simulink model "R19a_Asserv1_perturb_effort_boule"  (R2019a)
settings: Solver=ode15s  StartTime=0.0  StopTime=1  RelTol=1e-3  EnableMultiTasking=on
undefined symbols (not defined in the file): deg, kg, m, manette1_Défaut_sldprt, manette2_Défaut_sldprt, mm, N, rad, s, sigbuilder_block, STL, X, Y, Z
libraries: sm_lib x460, fl_lib x45, nesl_utility x23, simulink x3
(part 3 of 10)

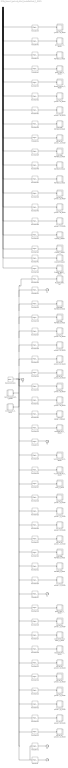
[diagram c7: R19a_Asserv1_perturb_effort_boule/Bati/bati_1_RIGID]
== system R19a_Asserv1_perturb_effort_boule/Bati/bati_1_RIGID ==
  CACHE_1_RIGID : Subsystem
  CACHE_2_RIGID : Subsystem
  CACHE_3_RIGID : Subsystem
  CARTER_ARRIERE_1_RIGID : Subsystem
  CARTE_HEXAGONALE_1_RIGID : Subsystem
  FIXATION_MOTEUR_1_RIGID : Subsystem
  FIXATION_MOTEUR_2_RIGID : Subsystem
  FIXATION_MOTEUR_3_RIGID : Subsystem
  FIXATION_MOTEUR_4_RIGID : Subsystem
  FIXATION_MOTEUR_5_RIGID : Subsystem
  FIXATION_MOTEUR_6_RIGID : Subsystem
  MOTEUR_1_RIGID : Subsystem
  MOTEUR_2_RIGID : Subsystem
  MOTEUR_3_RIGID : Subsystem
  PLAQUE_NOM_1_RIGID : Subsystem
  PLAQUE_NOM_SET : Subsystem
  ReferenceFrame : sm_lib/Frames and Transforms/Reference Frame
  Rondelle_M4_1_RIGID : Subsystem
  Rondelle_M4_2_RIGID : Subsystem
  Transform : sm_lib/Frames and Transforms/Rigid Transform  TranslationMethod=Cartesian  TranslationStandardOffset=0  TranslationLengthUnit=mm  TranslationStandardAxis=+Z  TranslationCartesianOffset=[-67.982453021745741 154.13917308955064 38.499999999999979]  TranslationROffset=0  TranslationROffsetUnits=m  TranslationZOffset=0  TranslationZOffsetUnits=m  TranslationThetaOffset=0  TranslationThetaOffsetUnits=deg  RotationMethod=ArbitraryAxis  RotationAngleUnits=rad  RotationStandardAxis=+Z  RotationAngle=2.2576709855630241  RotationArbitraryAxis=[-0.47317816576134769 -0.62293756647304832 0.62293756647304788]  FollAlignAxisA=+X  BaseAlignAxisA=+Y  FollAlignAxisB=+Y  BaseAlignAxisB=+Z  RotationSequenceAxes=FollowerAxes  RotationSequence=XYX  RotationSequenceAngles=[0 0 0]  RotationSequenceAnglesUnits=deg  RotationMatrix=[1 0 0; 0 1 0; 0 0 1]
  Transform1 : sm_lib/Frames and Transforms/Rigid Transform  TranslationMethod=Cartesian  TranslationStandardOffset=0  TranslationLengthUnit=mm  TranslationStandardAxis=+Z  TranslationCartesianOffset=[67.670238338594061 154.67994478363838 38.499999999999979]  TranslationROffset=0  TranslationROffsetUnits=m  TranslationZOffset=0  TranslationZOffsetUnits=m  TranslationThetaOffset=0  TranslationThetaOffsetUnits=deg  RotationMethod=ArbitraryAxis  RotationAngleUnits=rad  RotationStandardAxis=+Z  RotationAngle=2.2455218567975841  RotationArbitraryAxis=[-0.62007686508407689 -0.48063433374552811 -0.62007686508407622]  FollAlignAxisA=+X  BaseAlignAxisA=+Y  FollAlignAxisB=+Y  BaseAlignAxisB=+Z  RotationSequenceAxes=FollowerAxes  RotationSequence=XYX  RotationSequenceAngles=[0 0 0]  RotationSequenceAnglesUnits=deg  RotationMatrix=[1 0 0; 0 1 0; 0 0 1]
  Transform10 : sm_lib/Frames and Transforms/Rigid Transform  TranslationMethod=Cartesian  TranslationStandardOffset=0  TranslationLengthUnit=mm  TranslationStandardAxis=+Z  TranslationCartesianOffset=[-21.302011487444762 191.53150356202462 36.100000000000051]  TranslationROffset=0  TranslationROffsetUnits=m  TranslationZOffset=0  TranslationZOffsetUnits=m  TranslationThetaOffset=0  TranslationThetaOffsetUnits=deg  RotationMethod=ArbitraryAxis  RotationAngleUnits=rad  RotationStandardAxis=+Z  RotationAngle=1.5874169403231204  RotationArbitraryAxis=[0.12785986324311854 -0.98351599414696989 0.12785986324311688]  FollAlignAxisA=+X  BaseAlignAxisA=+Y  FollAlignAxisB=+Y  BaseAlignAxisB=+Z  RotationSequenceAxes=FollowerAxes  RotationSequence=XYX  RotationSequenceAngles=[0 0 0]  RotationSequenceAnglesUnits=deg  RotationMatrix=[1 0 0; 0 1 0; 0 0 1]
  Transform11 : sm_lib/Frames and Transforms/Rigid Transform  TranslationMethod=Cartesian  TranslationStandardOffset=0  TranslationLengthUnit=mm  TranslationStandardAxis=+Z  TranslationCartesianOffset=[-8.6943864691458312 146.25405010671241 36.099999999999994]  TranslationROffset=0  TranslationROffsetUnits=m  TranslationZOffset=0  TranslationZOffsetUnits=m  TranslationThetaOffset=0  TranslationThetaOffsetUnits=deg  RotationMethod=ArbitraryAxis  RotationAngleUnits=rad  RotationStandardAxis=+Z  RotationAngle=2.557922199918194  RotationArbitraryAxis=[0.67444507075713422 -0.30041253812517366 0.67444507075713389]  FollAlignAxisA=+X  BaseAlignAxisA=+Y  FollAlignAxisB=+Y  BaseAlignAxisB=+Z  RotationSequenceAxes=FollowerAxes  RotationSequence=XYX  RotationSequenceAngles=[0 0 0]  RotationSequenceAnglesUnits=deg  RotationMatrix=[1 0 0; 0 1 0; 0 0 1]
  Transform12 : sm_lib/Frames and Transforms/Rigid Transform  TranslationMethod=Cartesian  TranslationStandardOffset=0  TranslationLengthUnit=mm  TranslationStandardAxis=+Z  TranslationCartesianOffset=[31.197488247191473 107.27753449924363 36.099999999999994]  TranslationROffset=0  TranslationROffsetUnits=m  TranslationZOffset=0  TranslationZOffsetUnits=m  TranslationThetaOffset=0  TranslationThetaOffsetUnits=deg  RotationMethod=ArbitraryAxis  RotationAngleUnits=rad  RotationStandardAxis=+Z  RotationAngle=1.5816892610060764  RotationArbitraryAxis=[0.10380436397422958 -0.98916596587216399 0.10380436397423064]  FollAlignAxisA=+X  BaseAlignAxisA=+Y  FollAlignAxisB=+Y  BaseAlignAxisB=+Z  RotationSequenceAxes=FollowerAxes  RotationSequence=XYX  RotationSequenceAngles=[0 0 0]  RotationSequenceAnglesUnits=deg  RotationMatrix=[1 0 0; 0 1 0; 0 0 1]
  Transform13 : sm_lib/Frames and Transforms/Rigid Transform  TranslationMethod=Cartesian  TranslationStandardOffset=0  TranslationLengthUnit=mm  TranslationStandardAxis=+Z  TranslationCartesianOffset=[-32.1104315373926 141.51053427005223 49.100000000000001]  TranslationROffset=0  TranslationROffsetUnits=m  TranslationZOffset=0  TranslationZOffsetUnits=m  TranslationThetaOffset=0  TranslationThetaOffsetUnits=deg  RotationMethod=ArbitraryAxis  RotationAngleUnits=rad  RotationStandardAxis=+Z  RotationAngle=2.4188584057763718  RotationArbitraryAxis=[-0.65465367070797598 -0.37796447300923064 -0.6546536707079762]  FollAlignAxisA=+X  BaseAlignAxisA=+Y  FollAlignAxisB=+Y  BaseAlignAxisB=+Z  RotationSequenceAxes=FollowerAxes  RotationSequence=XYX  RotationSequenceAngles=[0 0 0]  RotationSequenceAnglesUnits=deg  RotationMatrix=[1 0 0; 0 1 0; 0 0 1]
  Transform14 : sm_lib/Frames and Transforms/Rigid Transform  TranslationMethod=Cartesian  TranslationStandardOffset=0  TranslationLengthUnit=mm  TranslationStandardAxis=+Z  TranslationCartesianOffset=[76.71272566730876 95.557331318822435 36.100000000000051]  TranslationROffset=0  TranslationROffsetUnits=m  TranslationZOffset=0  TranslationZOffsetUnits=m  TranslationThetaOffset=0  TranslationThetaOffsetUnits=deg  RotationMethod=ArbitraryAxis  RotationAngleUnits=rad  RotationStandardAxis=+Z  RotationAngle=2.253606277940353  RotationArbitraryAxis=[-0.62198874395633519 -0.47566795643940651 -0.62198874395633508]  FollAlignAxisA=+X  BaseAlignAxisA=+Y  FollAlignAxisB=+Y  BaseAlignAxisB=+Z  RotationSequenceAxes=FollowerAxes  RotationSequence=XYX  RotationSequenceAngles=[0 0 0]  RotationSequenceAnglesUnits=deg  RotationMatrix=[1 0 0; 0 1 0; 0 0 1]
  Transform15 : sm_lib/Frames and Transforms/Rigid Transform  TranslationMethod=Cartesian  TranslationStandardOffset=0  TranslationLengthUnit=mm  TranslationStandardAxis=+Z  TranslationCartesianOffset=[39.05251803832482 137.78242766379034 36.099999999999966]  TranslationROffset=0  TranslationROffsetUnits=m  TranslationZOffset=0  TranslationZOffsetUnits=m  TranslationThetaOffset=0  TranslationThetaOffsetUnits=deg  RotationMethod=ArbitraryAxis  RotationAngleUnits=rad  RotationStandardAxis=+Z  RotationAngle=2.1395291955010958  RotationArbitraryAxis=[-0.59164485304725056 -0.54764289069191197 -0.59164485304725156]  FollAlignAxisA=+X  BaseAlignAxisA=+Y  FollAlignAxisB=+Y  BaseAlignAxisB=+Z  RotationSequenceAxes=FollowerAxes  RotationSequence=XYX  RotationSequenceAngles=[0 0 0]  RotationSequenceAnglesUnits=deg  RotationMatrix=[1 0 0; 0 1 0; 0 0 1]
  Transform16 : sm_lib/Frames and Transforms/Rigid Transform  TranslationMethod=Cartesian  TranslationStandardOffset=0  TranslationLengthUnit=mm  TranslationStandardAxis=+Z  TranslationCartesianOffset=[-9.8750000000000053 1.2000000000000066 14.050000000000008]  TranslationROffset=0  TranslationROffsetUnits=m  TranslationZOffset=0  TranslationZOffsetUnits=m  TranslationThetaOffset=0  TranslationThetaOffsetUnits=deg  RotationMethod=ArbitraryAxis  RotationAngleUnits=rad  RotationStandardAxis=+Z  RotationAngle=0.1305039651717789  RotationArbitraryAxis=[1.6038157489539324e-15 1 -1.2797090690177757e-15]  FollAlignAxisA=+X  BaseAlignAxisA=+Y  FollAlignAxisB=+Y  BaseAlignAxisB=+Z  RotationSequenceAxes=FollowerAxes  RotationSequence=XYX  RotationSequenceAngles=[0 0 0]  RotationSequenceAnglesUnits=deg  RotationMatrix=[1 0 0; 0 1 0; 0 0 1]
  Transform17 : sm_lib/Frames and Transforms/Rigid Transform  TranslationMethod=Cartesian  TranslationStandardOffset=0  TranslationLengthUnit=mm  TranslationStandardAxis=+Z  TranslationCartesianOffset=[0 115.25000000000001 16.899999999999999]  TranslationROffset=0  TranslationROffsetUnits=m  TranslationZOffset=0  TranslationZOffsetUnits=m  TranslationThetaOffset=0  TranslationThetaOffsetUnits=deg  RotationMethod=ArbitraryAxis  RotationAngleUnits=rad  RotationStandardAxis=+Z  RotationAngle=3.1415926535897931  RotationArbitraryAxis=[-0.14780941112961105 0.98901586336191671 0]  FollAlignAxisA=+X  BaseAlignAxisA=+Y  FollAlignAxisB=+Y  BaseAlignAxisB=+Z  RotationSequenceAxes=FollowerAxes  RotationSequence=XYX  RotationSequenceAngles=[0 0 0]  RotationSequenceAnglesUnits=deg  RotationMatrix=[1 0 0; 0 1 0; 0 0 1]
  Transform18 : sm_lib/Frames and Transforms/Rigid Transform  TranslationMethod=Cartesian  TranslationStandardOffset=0  TranslationLengthUnit=mm  TranslationStandardAxis=+Z  TranslationCartesianOffset=[0 115.25000000000001 -1.799999999999996]  TranslationROffset=0  TranslationROffsetUnits=m  TranslationZOffset=0  TranslationZOffsetUnits=m  TranslationThetaOffset=0  TranslationThetaOffsetUnits=deg  RotationMethod=ArbitraryAxis  RotationAngleUnits=rad  RotationStandardAxis=+Z  RotationAngle=3.1415926535897909  RotationArbitraryAxis=[-0.70710678118654757 -1.2168216554799258e-15 -0.70710678118654746]  FollAlignAxisA=+X  BaseAlignAxisA=+Y  FollAlignAxisB=+Y  BaseAlignAxisB=+Z  RotationSequenceAxes=FollowerAxes  RotationSequence=XYX  RotationSequenceAngles=[0 0 0]  RotationSequenceAnglesUnits=deg  RotationMatrix=[1 0 0; 0 1 0; 0 0 1]
  Transform19 : sm_lib/Frames and Transforms/Rigid Transform  TranslationMethod=Cartesian  TranslationStandardOffset=0  TranslationLengthUnit=mm  TranslationStandardAxis=+Z  TranslationCartesianOffset=[-5.4923264138695282 106.15877278095202 52.900000000000013]  TranslationROffset=0  TranslationROffsetUnits=m  TranslationZOffset=0  TranslationZOffsetUnits=m  TranslationThetaOffset=0  TranslationThetaOffsetUnits=deg  RotationMethod=ArbitraryAxis  RotationAngleUnits=rad  RotationStandardAxis=+Z  RotationAngle=3.1415926535897931  RotationArbitraryAxis=[-0.62251463663761875 0.78260815685241447 9.5278235956943858e-17]  FollAlignAxisA=+X  BaseAlignAxisA=+Y  FollAlignAxisB=+Y  BaseAlignAxisB=+Z  RotationSequenceAxes=FollowerAxes  RotationSequence=XYX  RotationSequenceAngles=[0 0 0]  RotationSequenceAnglesUnits=deg  RotationMatrix=[1 0 0; 0 1 0; 0 0 1]
  Transform2 : sm_lib/Frames and Transforms/Rigid Transform  TranslationMethod=Cartesian  TranslationStandardOffset=0  TranslationLengthUnit=mm  TranslationStandardAxis=+Z  TranslationCartesianOffset=[0.3122146831511497 36.930882126810701 38.499999999999979]  TranslationROffset=0  TranslationROffsetUnits=m  TranslationZOffset=0  TranslationZOffsetUnits=m  TranslationThetaOffset=0  TranslationThetaOffsetUnits=deg  RotationMethod=ArbitraryAxis  RotationAngleUnits=rad  RotationStandardAxis=+Z  RotationAngle=1.7212826903554606  RotationArbitraryAxis=[0.85979818153437826 0.36107276761767659 0.36107276761767548]  FollAlignAxisA=+X  BaseAlignAxisA=+Y  FollAlignAxisB=+Y  BaseAlignAxisB=+Z  RotationSequenceAxes=FollowerAxes  RotationSequence=XYX  RotationSequenceAngles=[0 0 0]  RotationSequenceAnglesUnits=deg  RotationMatrix=[1 0 0; 0 1 0; 0 0 1]
  Transform20 : sm_lib/Frames and Transforms/Rigid Transform  TranslationMethod=Cartesian  TranslationStandardOffset=0  TranslationLengthUnit=mm  TranslationStandardAxis=+Z  TranslationCartesianOffset=[-6.6870740261211532 74.311283427110965 49.100000000000001]  TranslationROffset=0  TranslationROffsetUnits=m  TranslationZOffset=0  TranslationZOffsetUnits=m  TranslationThetaOffset=0  TranslationThetaOffsetUnits=deg  RotationMethod=ArbitraryAxis  RotationAngleUnits=rad  RotationStandardAxis=+Z  RotationAngle=1.5707963267948968  RotationArbitraryAxis=[-0 -1 -1.8723979605913744e-16]  FollAlignAxisA=+X  BaseAlignAxisA=+Y  FollAlignAxisB=+Y  BaseAlignAxisB=+Z  RotationSequenceAxes=FollowerAxes  RotationSequence=XYX  RotationSequenceAngles=[0 0 0]  RotationSequenceAnglesUnits=deg  RotationMatrix=[1 0 0; 0 1 0; 0 0 1]
  Transform21 : sm_lib/Frames and Transforms/Rigid Transform  TranslationMethod=Cartesian  TranslationStandardOffset=0  TranslationLengthUnit=mm  TranslationStandardAxis=+Z  TranslationCartesianOffset=[-16.466410454294302 53.38468832772007 38.500000000000007]  TranslationROffset=0  TranslationROffsetUnits=m  TranslationZOffset=0  TranslationZOffsetUnits=m  TranslationThetaOffset=0  TranslationThetaOffsetUnits=deg  RotationMethod=ArbitraryAxis  RotationAngleUnits=rad  RotationStandardAxis=+Z  RotationAngle=2.5869353710023297  RotationArbitraryAxis=[-0.28466429222446077 0.67785184248932562 -0.6778518424893254]  FollAlignAxisA=+X  BaseAlignAxisA=+Y  FollAlignAxisB=+Y  BaseAlignAxisB=+Z  RotationSequenceAxes=FollowerAxes  RotationSequence=XYX  RotationSequenceAngles=[0 0 0]  RotationSequenceAnglesUnits=deg  RotationMatrix=[1 0 0; 0 1 0; 0 0 1]
  Transform22 : sm_lib/Frames and Transforms/Rigid Transform  TranslationMethod=Cartesian  TranslationStandardOffset=0  TranslationLengthUnit=mm  TranslationStandardAxis=+Z  TranslationCartesianOffset=[-38.956907978955229 75.439790256598585 38.500000000000028]  TranslationROffset=0  TranslationROffsetUnits=m  TranslationZOffset=0  TranslationZOffsetUnits=m  TranslationThetaOffset=0  TranslationThetaOffsetUnits=deg  RotationMethod=ArbitraryAxis  RotationAngleUnits=rad  RotationStandardAxis=+Z  RotationAngle=2.5869353710023297  RotationArbitraryAxis=[-0.28466429222446077 0.67785184248932562 -0.67785184248932528]  FollAlignAxisA=+X  BaseAlignAxisA=+Y  FollAlignAxisB=+Y  BaseAlignAxisB=+Z  RotationSequenceAxes=FollowerAxes  RotationSequence=XYX  RotationSequenceAngles=[0 0 0]  RotationSequenceAnglesUnits=deg  RotationMatrix=[1 0 0; 0 1 0; 0 0 1]
  Transform23 : sm_lib/Frames and Transforms/Rigid Transform  TranslationMethod=Cartesian  TranslationStandardOffset=0  TranslationLengthUnit=mm  TranslationStandardAxis=+Z  TranslationCartesianOffset=[-32.920216655203667 36.606063190274597 36.100000000000037]  TranslationROffset=0  TranslationROffsetUnits=m  TranslationZOffset=0  TranslationZOffsetUnits=m  TranslationThetaOffset=0  TranslationThetaOffsetUnits=deg  RotationMethod=ArbitraryAxis  RotationAngleUnits=rad  RotationStandardAxis=+Z  RotationAngle=2.1079572963404796  RotationArbitraryAxis=[0.58180115951651357 -0.56834392894662011 0.58180115951651357]  FollAlignAxisA=+X  BaseAlignAxisA=+Y  FollAlignAxisB=+Y  BaseAlignAxisB=+Z  RotationSequenceAxes=FollowerAxes  RotationSequence=XYX  RotationSequenceAngles=[0 0 0]  RotationSequenceAnglesUnits=deg  RotationMatrix=[1 0 0; 0 1 0; 0 0 1]
  Transform24 : sm_lib/Frames and Transforms/Rigid Transform  TranslationMethod=Cartesian  TranslationStandardOffset=0  TranslationLengthUnit=mm  TranslationStandardAxis=+Z  TranslationCartesianOffset=[-55.410714179864605 58.661165119153118 36.100000000000051]  TranslationROffset=0  TranslationROffsetUnits=m  TranslationZOffset=0  TranslationZOffsetUnits=m  TranslationThetaOffset=0  TranslationThetaOffsetUnits=deg  RotationMethod=ArbitraryAxis  RotationAngleUnits=rad  RotationStandardAxis=+Z  RotationAngle=2.5913633997650876  RotationArbitraryAxis=[0.67835179231251819 -0.28227237153641171 0.67835179231251697]  FollAlignAxisA=+X  BaseAlignAxisA=+Y  FollAlignAxisB=+Y  BaseAlignAxisB=+Z  RotationSequenceAxes=FollowerAxes  RotationSequence=XYX  RotationSequenceAngles=[0 0 0]  RotationSequenceAnglesUnits=deg  RotationMatrix=[1 0 0; 0 1 0; 0 0 1]
  Transform25 : sm_lib/Frames and Transforms/Rigid Transform  TranslationMethod=Cartesian  TranslationStandardOffset=0  TranslationLengthUnit=mm  TranslationStandardAxis=+Z  TranslationCartesianOffset=[-0.012604253384927124 70.163313465165515 36.099999999999966]  TranslationROffset=0  TranslationROffsetUnits=m  TranslationZOffset=0  TranslationZOffsetUnits=m  TranslationThetaOffset=0  TranslationThetaOffsetUnits=deg  RotationMethod=ArbitraryAxis  RotationAngleUnits=rad  RotationStandardAxis=+Z  RotationAngle=2.7200049334585095  RotationArbitraryAxis=[0.6907299635194234 -0.21397250990001554 0.6907299635194234]  FollAlignAxisA=+X  BaseAlignAxisA=+Y  FollAlignAxisB=+Y  BaseAlignAxisB=+Z  RotationSequenceAxes=FollowerAxes  RotationSequence=XYX  RotationSequenceAngles=[0 0 0]  RotationSequenceAnglesUnits=deg  RotationMatrix=[1 0 0; 0 1 0; 0 0 1]
  Transform26 : sm_lib/Frames and Transforms/Rigid Transform  TranslationMethod=Cartesian  TranslationStandardOffset=0  TranslationLengthUnit=mm  TranslationStandardAxis=+Z  TranslationCartesianOffset=[-22.503101778045874 92.21841539404403 36.099999999999994]  TranslationROffset=0  TranslationROffsetUnits=m  TranslationZOffset=0  TranslationZOffsetUnits=m  TranslationThetaOffset=0  TranslationThetaOffsetUnits=deg  RotationMethod=ArbitraryAxis  RotationAngleUnits=rad  RotationStandardAxis=+Z  RotationAngle=2.2845314039372839  RotationArbitraryAxis=[-0.62900467206978528 -0.4568437862429186 -0.62900467206978417]  FollAlignAxisA=+X  BaseAlignAxisA=+Y  FollAlignAxisB=+Y  BaseAlignAxisB=+Z  RotationSequenceAxes=FollowerAxes  RotationSequence=XYX  RotationSequenceAngles=[0 0 0]  RotationSequenceAnglesUnits=deg  RotationMatrix=[1 0 0; 0 1 0; 0 0 1]
  Transform27 : sm_lib/Frames and Transforms/Rigid Transform  TranslationMethod=Cartesian  TranslationStandardOffset=0  TranslationLengthUnit=mm  TranslationStandardAxis=+Z  TranslationCartesianOffset=[0 -1.5000000000000151 37.700000000000003]  TranslationROffset=0  TranslationROffsetUnits=m  TranslationZOffset=0  TranslationZOffsetUnits=m  TranslationThetaOffset=0  TranslationThetaOffsetUnits=deg  RotationMethod=ArbitraryAxis  RotationAngleUnits=rad  RotationStandardAxis=+Z  RotationAngle=1.5707963267948961  RotationArbitraryAxis=[-1 0 0]  FollAlignAxisA=+X  BaseAlignAxisA=+Y  FollAlignAxisB=+Y  BaseAlignAxisB=+Z  RotationSequenceAxes=FollowerAxes  RotationSequence=XYX  RotationSequenceAngles=[0 0 0]  RotationSequenceAnglesUnits=deg  RotationMatrix=[1 0 0; 0 1 0; 0 0 1]
  Transform28 : sm_lib/Frames and Transforms/Rigid Transform  TranslationMethod=Cartesian  TranslationStandardOffset=0  TranslationLengthUnit=mm  TranslationStandardAxis=+Z  TranslationCartesianOffset=[9.8750000000000089 31.199999999999992 14.050000000000008]  TranslationROffset=0  TranslationROffsetUnits=m  TranslationZOffset=0  TranslationZOffsetUnits=m  TranslationThetaOffset=0  TranslationThetaOffsetUnits=deg  RotationMethod=ArbitraryAxis  RotationAngleUnits=rad  RotationStandardAxis=+Z  RotationAngle=2.773492570857111  RotationArbitraryAxis=[0.18615678789738549 -0.69474659060686594 0.69474659060686572]  FollAlignAxisA=+X  BaseAlignAxisA=+Y  FollAlignAxisB=+Y  BaseAlignAxisB=+Z  RotationSequenceAxes=FollowerAxes  RotationSequence=XYX  RotationSequenceAngles=[0 0 0]  RotationSequenceAnglesUnits=deg  RotationMatrix=[1 0 0; 0 1 0; 0 0 1]
  Transform29 : sm_lib/Frames and Transforms/Rigid Transform  TranslationMethod=Cartesian  TranslationStandardOffset=0  TranslationLengthUnit=mm  TranslationStandardAxis=+Z  TranslationCartesianOffset=[-9.8750000000000053 31.199999999999992 14.050000000000008]  TranslationROffset=0  TranslationROffsetUnits=m  TranslationZOffset=0  TranslationZOffsetUnits=m  TranslationThetaOffset=0  TranslationThetaOffsetUnits=deg  RotationMethod=ArbitraryAxis  RotationAngleUnits=rad  RotationStandardAxis=+Z  RotationAngle=2.773492570857111  RotationArbitraryAxis=[0.18615678789738549 -0.69474659060686594 0.69474659060686572]  FollAlignAxisA=+X  BaseAlignAxisA=+Y  FollAlignAxisB=+Y  BaseAlignAxisB=+Z  RotationSequenceAxes=FollowerAxes  RotationSequence=XYX  RotationSequenceAngles=[0 0 0]  RotationSequenceAnglesUnits=deg  RotationMatrix=[1 0 0; 0 1 0; 0 0 1]
  Transform3 : sm_lib/Frames and Transforms/Rigid Transform  TranslationMethod=Cartesian  TranslationStandardOffset=0  TranslationLengthUnit=mm  TranslationStandardAxis=+Z  TranslationCartesianOffset=[-106.82639785458468 167.86430788780581 99.318100970001225]  TranslationROffset=0  TranslationROffsetUnits=m  TranslationZOffset=0  TranslationZOffsetUnits=m  TranslationThetaOffset=0  TranslationThetaOffsetUnits=deg  RotationMethod=ArbitraryAxis  RotationAngleUnits=rad  RotationStandardAxis=+Z  RotationAngle=1.7212826903554632  RotationArbitraryAxis=[0.85979818153438259 0.36107276761767909 0.36107276761766205]  FollAlignAxisA=+X  BaseAlignAxisA=+Y  FollAlignAxisB=+Y  BaseAlignAxisB=+Z  RotationSequenceAxes=FollowerAxes  RotationSequence=XYX  RotationSequenceAngles=[0 0 0]  RotationSequenceAnglesUnits=deg  RotationMatrix=[1 0 0; 0 1 0; 0 0 1]
  Transform30 : sm_lib/Frames and Transforms/Rigid Transform  TranslationMethod=Cartesian  TranslationStandardOffset=0  TranslationLengthUnit=mm  TranslationStandardAxis=+Z  TranslationCartesianOffset=[9.8750000000000089 2.0000000000000018 14.050000000000008]  TranslationROffset=0  TranslationROffsetUnits=m  TranslationZOffset=0  TranslationZOffsetUnits=m  TranslationThetaOffset=0  TranslationThetaOffsetUnits=deg  RotationMethod=ArbitraryAxis  RotationAngleUnits=rad  RotationStandardAxis=+Z  RotationAngle=3.1415926535897931  RotationArbitraryAxis=[-0.99787184465383982 -0 0.065205687230048659]  FollAlignAxisA=+X  BaseAlignAxisA=+Y  FollAlignAxisB=+Y  BaseAlignAxisB=+Z  RotationSequenceAxes=FollowerAxes  RotationSequence=XYX  RotationSequenceAngles=[0 0 0]  RotationSequenceAnglesUnits=deg  RotationMatrix=[1 0 0; 0 1 0; 0 0 1]
  Transform31 : sm_lib/Frames and Transforms/Rigid Transform  TranslationMethod=None  TranslationStandardOffset=0  TranslationLengthUnit=m  TranslationStandardAxis=+Z  TranslationCartesianOffset=[0 0 0]  TranslationROffset=0  TranslationROffsetUnits=m  TranslationZOffset=0  TranslationZOffsetUnits=m  TranslationThetaOffset=0  TranslationThetaOffsetUnits=deg  RotationMethod=ArbitraryAxis  RotationAngleUnits=rad  RotationStandardAxis=+Z  RotationAngle=3.1415926535897931  RotationArbitraryAxis=[0 1 0]  FollAlignAxisA=+X  BaseAlignAxisA=+Y  FollAlignAxisB=+Y  BaseAlignAxisB=+Z  RotationSequenceAxes=FollowerAxes  RotationSequence=XYX  RotationSequenceAngles=[0 0 0]  RotationSequenceAnglesUnits=deg  RotationMatrix=[1 0 0; 0 1 0; 0 0 1]
  Transform32 : sm_lib/Frames and Transforms/Rigid Transform  TranslationMethod=Cartesian  TranslationStandardOffset=0  TranslationLengthUnit=mm  TranslationStandardAxis=+Z  TranslationCartesianOffset=[78.177113545509911 88.894999319852587 19.199999999999996]  TranslationROffset=0  TranslationROffsetUnits=m  TranslationZOffset=0  TranslationZOffsetUnits=m  TranslationThetaOffset=0  TranslationThetaOffsetUnits=deg  RotationMethod=ArbitraryAxis  RotationAngleUnits=rad  RotationStandardAxis=+Z  RotationAngle=1.6591931073504684  RotationArbitraryAxis=[-0.28481620059537222 -0.91529201010214944 -0.28481620059537222]  FollAlignAxisA=+X  BaseAlignAxisA=+Y  FollAlignAxisB=+Y  BaseAlignAxisB=+Z  RotationSequenceAxes=FollowerAxes  RotationSequence=XYX  RotationSequenceAngles=[0 0 0]  RotationSequenceAnglesUnits=deg  RotationMatrix=[1 0 0; 0 1 0; 0 0 1]
  Transform33 : sm_lib/Frames and Transforms/Rigid Transform  TranslationMethod=Cartesian  TranslationStandardOffset=0  TranslationLengthUnit=mm  TranslationStandardAxis=+Z  TranslationCartesianOffset=[56.590549141302901 55.218676943733961 19.199999999999996]  TranslationROffset=0  TranslationROffsetUnits=m  TranslationZOffset=0  TranslationZOffsetUnits=m  TranslationThetaOffset=0  TranslationThetaOffsetUnits=deg  RotationMethod=ArbitraryAxis  RotationAngleUnits=rad  RotationStandardAxis=+Z  RotationAngle=1.5707963267948968  RotationArbitraryAxis=[-0 -1 -0]  FollAlignAxisA=+X  BaseAlignAxisA=+Y  FollAlignAxisB=+Y  BaseAlignAxisB=+Z  RotationSequenceAxes=FollowerAxes  RotationSequence=XYX  RotationSequenceAngles=[0 0 0]  RotationSequenceAnglesUnits=deg  RotationMatrix=[1 0 0; 0 1 0; 0 0 1]
  Transform34 : sm_lib/Frames and Transforms/Rigid Transform  TranslationMethod=Cartesian  TranslationStandardOffset=0  TranslationLengthUnit=mm  TranslationStandardAxis=+Z  TranslationCartesianOffset=[23.693376218865065 194.27451469861313 19.199999999999996]  TranslationROffset=0  TranslationROffsetUnits=m  TranslationZOffset=0  TranslationZOffsetUnits=m  TranslationThetaOffset=0  TranslationThetaOffsetUnits=deg  RotationMethod=ArbitraryAxis  RotationAngleUnits=rad  RotationStandardAxis=+Z  RotationAngle=2.4188584057763807  RotationArbitraryAxis=[0.65465367070797764 -0.37796447300922553 0.65465367070797764]  FollAlignAxisA=+X  BaseAlignAxisA=+Y  FollAlignAxisB=+Y  BaseAlignAxisB=+Z  RotationSequenceAxes=FollowerAxes  RotationSequence=XYX  RotationSequenceAngles=[0 0 0]  RotationSequenceAnglesUnits=deg  RotationMatrix=[1 0 0; 0 1 0; 0 0 1]
  Transform35 : sm_lib/Frames and Transforms/Rigid Transform  TranslationMethod=Cartesian  TranslationStandardOffset=0  TranslationLengthUnit=mm  TranslationStandardAxis=+Z  TranslationCartesianOffset=[-80.283925360168155 96.256808357652318 19.199999999999996]  TranslationROffset=0  TranslationROffsetUnits=m  TranslationZOffset=0  TranslationZOffsetUnits=m  TranslationThetaOffset=0  TranslationThetaOffsetUnits=deg  RotationMethod=ArbitraryAxis  RotationAngleUnits=rad  RotationStandardAxis=+Z  RotationAngle=2.4188584057763718  RotationArbitraryAxis=[-0.65465367070797598 -0.37796447300923064 -0.65465367070797609]  FollAlignAxisA=+X  BaseAlignAxisA=+Y  FollAlignAxisB=+Y  BaseAlignAxisB=+Z  RotationSequenceAxes=FollowerAxes  RotationSequence=XYX  RotationSequenceAngles=[0 0 0]  RotationSequenceAnglesUnits=deg  RotationMatrix=[1 0 0; 0 1 0; 0 0 1]
  Transform36 : sm_lib/Frames and Transforms/Rigid Transform  TranslationMethod=Cartesian  TranslationStandardOffset=0  TranslationLengthUnit=mm  TranslationStandardAxis=+Z  TranslationCartesianOffset=[-16.264456666991514 196.13086666502576 19.199999999999996]  TranslationROffset=0  TranslationROffsetUnits=m  TranslationZOffset=0  TranslationZOffsetUnits=m  TranslationThetaOffset=0  TranslationThetaOffsetUnits=deg  RotationMethod=ArbitraryAxis  RotationAngleUnits=rad  RotationStandardAxis=+Z  RotationAngle=2.0489764020053052  RotationArbitraryAxis=[0.56137820698022478 -0.60803701980663627 0.56137820698022478]  FollAlignAxisA=+X  BaseAlignAxisA=+Y  FollAlignAxisB=+Y  BaseAlignAxisB=+Z  RotationSequenceAxes=FollowerAxes  RotationSequence=XYX  RotationSequenceAngles=[0 0 0]  RotationSequenceAnglesUnits=deg  RotationMatrix=[1 0 0; 0 1 0; 0 0 1]
  Transform37 : sm_lib/Frames and Transforms/Rigid Transform  TranslationMethod=Cartesian  TranslationStandardOffset=0  TranslationLengthUnit=mm  TranslationStandardAxis=+Z  TranslationCartesianOffset=[-61.912656878518263 60.724134015121031 19.199999999999996]  TranslationROffset=0  TranslationROffsetUnits=m  TranslationZOffset=0  TranslationZOffsetUnits=m  TranslationThetaOffset=0  TranslationThetaOffsetUnits=deg  RotationMethod=ArbitraryAxis  RotationAngleUnits=rad  RotationStandardAxis=+Z  RotationAngle=2.8290477720117608  RotationArbitraryAxis=[-0.69827493103712956 -0.15755710510854135 -0.69827493103712956]  FollAlignAxisA=+X  BaseAlignAxisA=+Y  FollAlignAxisB=+Y  BaseAlignAxisB=+Z  RotationSequenceAxes=FollowerAxes  RotationSequence=XYX  RotationSequenceAngles=[0 0 0]  RotationSequenceAnglesUnits=deg  RotationMatrix=[1 0 0; 0 1 0; 0 0 1]
  Transform38 : sm_lib/Frames and Transforms/Rigid Transform  TranslationMethod=Cartesian  TranslationStandardOffset=0  TranslationLengthUnit=mm  TranslationStandardAxis=+Z  TranslationCartesianOffset=[61.810136748383464 131.92232607357974 38.500000000000007]  TranslationROffset=0  TranslationROffsetUnits=m  TranslationZOffset=0  TranslationZOffsetUnits=m  TranslationThetaOffset=0  TranslationThetaOffsetUnits=deg  RotationMethod=ArbitraryAxis  RotationAngleUnits=rad  RotationStandardAxis=+Z  RotationAngle=1.5865923302678127  RotationArbitraryAxis=[-0.98432745245712761 0.12469856923650155 -0.1246985692365027]  FollAlignAxisA=+X  BaseAlignAxisA=+Y  FollAlignAxisB=+Y  BaseAlignAxisB=+Z  RotationSequenceAxes=FollowerAxes  RotationSequence=XYX  RotationSequenceAngles=[0 0 0]  RotationSequenceAnglesUnits=deg  RotationMatrix=[1 0 0; 0 1 0; 0 0 1]
  Transform39 : sm_lib/Frames and Transforms/Rigid Transform  TranslationMethod=Cartesian  TranslationStandardOffset=0  TranslationLengthUnit=mm  TranslationStandardAxis=+Z  TranslationCartesianOffset=[-45.343726294089642 160.44298559870006 38.500000000000007]  TranslationROffset=0  TranslationROffsetUnits=m  TranslationZOffset=0  TranslationZOffsetUnits=m  TranslationThetaOffset=0  TranslationThetaOffsetUnits=deg  RotationMethod=ArbitraryAxis  RotationAngleUnits=rad  RotationStandardAxis=+Z  RotationAngle=2.2576709855630233  RotationArbitraryAxis=[-0.47317816576134747 -0.62293756647304876 0.62293756647304765]  FollAlignAxisA=+X  BaseAlignAxisA=+Y  FollAlignAxisB=+Y  BaseAlignAxisB=+Z  RotationSequenceAxes=FollowerAxes  RotationSequence=XYX  RotationSequenceAngles=[0 0 0]  RotationSequenceAnglesUnits=deg  RotationMatrix=[1 0 0; 0 1 0; 0 0 1]
  Transform4 : sm_lib/Frames and Transforms/Rigid Transform  TranslationMethod=Cartesian  TranslationStandardOffset=0  TranslationLengthUnit=mm  TranslationStandardAxis=+Z  TranslationCartesianOffset=[7.8478716939170852 -3.5715282807566169 99.318100970001225]  TranslationROffset=0  TranslationROffsetUnits=m  TranslationZOffset=0  TranslationZOffsetUnits=m  TranslationThetaOffset=0  TranslationThetaOffsetUnits=deg  RotationMethod=ArbitraryAxis  RotationAngleUnits=rad  RotationStandardAxis=+Z  RotationAngle=2.2455218567975974  RotationArbitraryAxis=[-0.62007686508408166 -0.48063433374552633 -0.62007686508407289]  FollAlignAxisA=+X  BaseAlignAxisA=+Y  FollAlignAxisB=+Y  BaseAlignAxisB=+Z  RotationSequenceAxes=FollowerAxes  RotationSequence=XYX  RotationSequenceAngles=[0 0 0]  RotationSequenceAnglesUnits=deg  RotationMatrix=[1 0 0; 0 1 0; 0 0 1]
  Transform40 : sm_lib/Frames and Transforms/Rigid Transform  TranslationMethod=Cartesian  TranslationStandardOffset=0  TranslationLengthUnit=mm  TranslationStandardAxis=+Z  TranslationCartesianOffset=[-30 40 75]  TranslationROffset=0  TranslationROffsetUnits=m  TranslationZOffset=0  TranslationZOffsetUnits=m  TranslationThetaOffset=0  TranslationThetaOffsetUnits=deg  RotationMethod=None  RotationAngleUnits=rad  RotationStandardAxis=+Z  RotationAngle=2.0835623886098844e-12  RotationArbitraryAxis=[1 0 0]  FollAlignAxisA=+X  BaseAlignAxisA=+Y  FollAlignAxisB=+Y  BaseAlignAxisB=+Z  RotationSequenceAxes=FollowerAxes  RotationSequence=XYX  RotationSequenceAngles=[0 0 0]  RotationSequenceAnglesUnits=deg  RotationMatrix=[1 0 0; 0 1 0; 0 0 1]
  Transform41 : sm_lib/Frames and Transforms/Rigid Transform  TranslationMethod=Cartesian  TranslationStandardOffset=0  TranslationLengthUnit=mm  TranslationStandardAxis=+Z  TranslationCartesianOffset=[-1.3156175645385466e-09 0 24.000000000062251]  TranslationROffset=0  TranslationROffsetUnits=m  TranslationZOffset=0  TranslationZOffsetUnits=m  TranslationThetaOffset=0  TranslationThetaOffsetUnits=deg  RotationMethod=ArbitraryAxis  RotationAngleUnits=rad  RotationStandardAxis=+Z  RotationAngle=1.1415336785562208e-11  RotationArbitraryAxis=[0 0 -1]  FollAlignAxisA=+X  BaseAlignAxisA=+Y  FollAlignAxisB=+Y  BaseAlignAxisB=+Z  RotationSequenceAxes=FollowerAxes  RotationSequence=XYX  RotationSequenceAngles=[0 0 0]  RotationSequenceAnglesUnits=deg  RotationMatrix=[1 0 0; 0 1 0; 0 0 1]
  Transform42 : sm_lib/Frames and Transforms/Rigid Transform  TranslationMethod=Cartesian  TranslationStandardOffset=0  TranslationLengthUnit=mm  TranslationStandardAxis=+Z  TranslationCartesianOffset=[99.809427786814155 172.87499999886114 24.000000000062251]  TranslationROffset=0  TranslationROffsetUnits=m  TranslationZOffset=0  TranslationZOffsetUnits=m  TranslationThetaOffset=0  TranslationThetaOffsetUnits=deg  RotationMethod=ArbitraryAxis  RotationAngleUnits=rad  RotationStandardAxis=+Z  RotationAngle=2.0943951023817848  RotationArbitraryAxis=[0 0 1]  FollAlignAxisA=+X  BaseAlignAxisA=+Y  FollAlignAxisB=+Y  BaseAlignAxisB=+Z  RotationSequenceAxes=FollowerAxes  RotationSequence=XYX  RotationSequenceAngles=[0 0 0]  RotationSequenceAnglesUnits=deg  RotationMatrix=[1 0 0; 0 1 0; 0 0 1]
  Transform43 : sm_lib/Frames and Transforms/Rigid Transform  TranslationMethod=Cartesian  TranslationStandardOffset=0  TranslationLengthUnit=mm  TranslationStandardAxis=+Z  TranslationCartesianOffset=[-99.809427785499309 172.87500000113846 24.000000000062251]  TranslationROffset=0  TranslationROffsetUnits=m  TranslationZOffset=0  TranslationZOffsetUnits=m  TranslationThetaOffset=0  TranslationThetaOffsetUnits=deg  RotationMethod=ArbitraryAxis  RotationAngleUnits=rad  RotationStandardAxis=+Z  RotationAngle=2.0943951024046012  RotationArbitraryAxis=[-0 -0 -1]  FollAlignAxisA=+X  BaseAlignAxisA=+Y  FollAlignAxisB=+Y  BaseAlignAxisB=+Z  RotationSequenceAxes=FollowerAxes  RotationSequence=XYX  RotationSequenceAngles=[0 0 0]  RotationSequenceAnglesUnits=deg  RotationMatrix=[1 0 0; 0 1 0; 0 0 1]
  Transform44 : sm_lib/Frames and Transforms/Rigid Transform  TranslationMethod=Cartesian  TranslationStandardOffset=0  TranslationLengthUnit=mm  TranslationStandardAxis=+Z  TranslationCartesianOffset=[13.533207794599599 64.174992098843177 13.600000000000001]  TranslationROffset=0  TranslationROffsetUnits=m  TranslationZOffset=0  TranslationZOffsetUnits=m  TranslationThetaOffset=0  TranslationThetaOffsetUnits=deg  RotationMethod=ArbitraryAxis  RotationAngleUnits=rad  RotationStandardAxis=+Z  RotationAngle=1.5707963267948968  RotationArbitraryAxis=[-0 -1 -0]  FollAlignAxisA=+X  BaseAlignAxisA=+Y  FollAlignAxisB=+Y  BaseAlignAxisB=+Z  RotationSequenceAxes=FollowerAxes  RotationSequence=XYX  RotationSequenceAngles=[0 0 0]  RotationSequenceAnglesUnits=deg  RotationMatrix=[1 0 0; 0 1 0; 0 0 1]
  Transform45 : sm_lib/Frames and Transforms/Rigid Transform  TranslationMethod=Cartesian  TranslationStandardOffset=0  TranslationLengthUnit=mm  TranslationStandardAxis=+Z  TranslationCartesianOffset=[84.567755458442107 126.06222448336912 36.100000000000037]  TranslationROffset=0  TranslationROffsetUnits=m  TranslationZOffset=0  TranslationZOffsetUnits=m  TranslationThetaOffset=0  TranslationThetaOffsetUnits=deg  RotationMethod=ArbitraryAxis  RotationAngleUnits=rad  RotationStandardAxis=+Z  RotationAngle=2.7572489937583149  RotationArbitraryAxis=[-0.69359259312433763 -0.19457294140273607 -0.69359259312433874]  FollAlignAxisA=+X  BaseAlignAxisA=+Y  FollAlignAxisB=+Y  BaseAlignAxisB=+Z  RotationSequenceAxes=FollowerAxes  RotationSequence=XYX  RotationSequenceAngles=[0 0 0]  RotationSequenceAnglesUnits=deg  RotationMatrix=[1 0 0; 0 1 0; 0 0 1]
  Transform46 : sm_lib/Frames and Transforms/Rigid Transform  TranslationMethod=Cartesian  TranslationStandardOffset=0  TranslationLengthUnit=mm  TranslationStandardAxis=+Z  TranslationCartesianOffset=[-51.647538803239108 183.08171232635618 36.100000000000037]  TranslationROffset=0  TranslationROffsetUnits=m  TranslationZOffset=0  TranslationZOffsetUnits=m  TranslationThetaOffset=0  TranslationThetaOffsetUnits=deg  RotationMethod=ArbitraryAxis  RotationAngleUnits=rad  RotationStandardAxis=+Z  RotationAngle=1.6320911114092145  RotationArbitraryAxis=[-0.24025122409678262 -0.94050980783827787 -0.24025122409678393]  FollAlignAxisA=+X  BaseAlignAxisA=+Y  FollAlignAxisB=+Y  BaseAlignAxisB=+Z  RotationSequenceAxes=FollowerAxes  RotationSequence=XYX  RotationSequenceAngles=[0 0 0]  RotationSequenceAnglesUnits=deg  RotationMatrix=[1 0 0; 0 1 0; 0 0 1]
  Transform47 : sm_lib/Frames and Transforms/Rigid Transform  TranslationMethod=Cartesian  TranslationStandardOffset=0  TranslationLengthUnit=mm  TranslationStandardAxis=+Z  TranslationCartesianOffset=[67.670238338594061 154.67994478363838 38.499999999999979]  TranslationROffset=0  TranslationROffsetUnits=m  TranslationZOffset=0  TranslationZOffsetUnits=m  TranslationThetaOffset=0  TranslationThetaOffsetUnits=deg  RotationMethod=ArbitraryAxis  RotationAngleUnits=rad  RotationStandardAxis=+Z  RotationAngle=3.1415926535897922  RotationArbitraryAxis=[0.99207089132052606 -0.125679539283437 6.6259454489207254e-17]  FollAlignAxisA=+X  BaseAlignAxisA=+Y  FollAlignAxisB=+Y  BaseAlignAxisB=+Z  RotationSequenceAxes=FollowerAxes  RotationSequence=XYX  RotationSequenceAngles=[0 0 0]  RotationSequenceAnglesUnits=deg  RotationMatrix=[1 0 0; 0 1 0; 0 0 1]
  Transform48 : sm_lib/Frames and Transforms/Rigid Transform  TranslationMethod=Cartesian  TranslationStandardOffset=0  TranslationLengthUnit=mm  TranslationStandardAxis=+Z  TranslationCartesianOffset=[-67.982453021745741 154.13917308955064 38.499999999999979]  TranslationROffset=0  TranslationROffsetUnits=m  TranslationZOffset=0  TranslationZOffsetUnits=m  TranslationThetaOffset=0  TranslationThetaOffsetUnits=deg  RotationMethod=ArbitraryAxis  RotationAngleUnits=rad  RotationStandardAxis=+Z  RotationAngle=3.1415926535897931  RotationArbitraryAxis=[0.60487711941564182 0.79631882459692971 4.2817701064170949e-16]  FollAlignAxisA=+X  BaseAlignAxisA=+Y  FollAlignAxisB=+Y  BaseAlignAxisB=+Z  RotationSequenceAxes=FollowerAxes  RotationSequence=XYX  RotationSequenceAngles=[0 0 0]  RotationSequenceAnglesUnits=deg  RotationMatrix=[1 0 0; 0 1 0; 0 0 1]
  Transform49 : sm_lib/Frames and Transforms/Rigid Transform  TranslationMethod=Cartesian  TranslationStandardOffset=0  TranslationLengthUnit=mm  TranslationStandardAxis=+Z  TranslationCartesianOffset=[53.955106957250102 101.41743290903302 38.500000000000028]  TranslationROffset=0  TranslationROffsetUnits=m  TranslationZOffset=0  TranslationZOffsetUnits=m  TranslationThetaOffset=0  TranslationThetaOffsetUnits=deg  RotationMethod=ArbitraryAxis  RotationAngleUnits=rad  RotationStandardAxis=+Z  RotationAngle=1.5865923302678127  RotationArbitraryAxis=[-0.98432745245712761 0.12469856923650148 -0.12469856923650251]  FollAlignAxisA=+X  BaseAlignAxisA=+Y  FollAlignAxisB=+Y  BaseAlignAxisB=+Z  RotationSequenceAxes=FollowerAxes  RotationSequence=XYX  RotationSequenceAngles=[0 0 0]  RotationSequenceAnglesUnits=deg  RotationMatrix=[1 0 0; 0 1 0; 0 0 1]
  Transform5 : sm_lib/Frames and Transforms/Rigid Transform  TranslationMethod=Cartesian  TranslationStandardOffset=0  TranslationLengthUnit=mm  TranslationStandardAxis=+Z  TranslationCartesianOffset=[38.79750556351344 129.92818230283672 49.100000000000001]  TranslationROffset=0  TranslationROffsetUnits=m  TranslationZOffset=0  TranslationZOffsetUnits=m  TranslationThetaOffset=0  TranslationThetaOffsetUnits=deg  RotationMethod=ArbitraryAxis  RotationAngleUnits=rad  RotationStandardAxis=+Z  RotationAngle=2.4188584057763802  RotationArbitraryAxis=[0.65465367070797764 -0.37796447300922548 0.65465367070797764]  FollAlignAxisA=+X  BaseAlignAxisA=+Y  FollAlignAxisB=+Y  BaseAlignAxisB=+Z  RotationSequenceAxes=FollowerAxes  RotationSequence=XYX  RotationSequenceAngles=[0 0 0]  RotationSequenceAnglesUnits=deg  RotationMatrix=[1 0 0; 0 1 0; 0 0 1]
  Transform50 : sm_lib/Frames and Transforms/Rigid Transform  TranslationMethod=Cartesian  TranslationStandardOffset=0  TranslationLengthUnit=mm  TranslationStandardAxis=+Z  TranslationCartesianOffset=[-14.998198978295296 168.8927768343685 38.500000000000028]  TranslationROffset=0  TranslationROffsetUnits=m  TranslationZOffset=0  TranslationZOffsetUnits=m  TranslationThetaOffset=0  TranslationThetaOffsetUnits=deg  RotationMethod=ArbitraryAxis  RotationAngleUnits=rad  RotationStandardAxis=+Z  RotationAngle=2.2576709855630233  RotationArbitraryAxis=[-0.47317816576134758 -0.62293756647304876 0.62293756647304777]  FollAlignAxisA=+X  BaseAlignAxisA=+Y  FollAlignAxisB=+Y  BaseAlignAxisB=+Z  RotationSequenceAxes=FollowerAxes  RotationSequence=XYX  RotationSequenceAngles=[0 0 0]  RotationSequenceAnglesUnits=deg  RotationMatrix=[1 0 0; 0 1 0; 0 0 1]
  Transform51 : sm_lib/Frames and Transforms/Rigid Transform  TranslationMethod=Cartesian  TranslationStandardOffset=0  TranslationLengthUnit=mm  TranslationStandardAxis=+Z  TranslationCartesianOffset=[37.465650443592779 152.50760569539543 13.600000000000001]  TranslationROffset=0  TranslationROffsetUnits=m  TranslationZOffset=0  TranslationZOffsetUnits=m  TranslationThetaOffset=0  TranslationThetaOffsetUnits=deg  RotationMethod=ArbitraryAxis  RotationAngleUnits=rad  RotationStandardAxis=+Z  RotationAngle=2.4188584057763807  RotationArbitraryAxis=[0.65465367070797775 -0.37796447300922559 0.65465367070797753]  FollAlignAxisA=+X  BaseAlignAxisA=+Y  FollAlignAxisB=+Y  BaseAlignAxisB=+Z  RotationSequenceAxes=FollowerAxes  RotationSequence=XYX  RotationSequenceAngles=[0 0 0]  RotationSequenceAnglesUnits=deg  RotationMatrix=[1 0 0; 0 1 0; 0 0 1]
  Transform52 : sm_lib/Frames and Transforms/Rigid Transform  TranslationMethod=Cartesian  TranslationStandardOffset=0  TranslationLengthUnit=mm  TranslationStandardAxis=+Z  TranslationCartesianOffset=[-50.998858238192668 129.06740220576114 13.600000000000001]  TranslationROffset=0  TranslationROffsetUnits=m  TranslationZOffset=0  TranslationZOffsetUnits=m  TranslationThetaOffset=0  TranslationThetaOffsetUnits=deg  RotationMethod=ArbitraryAxis  RotationAngleUnits=rad  RotationStandardAxis=+Z  RotationAngle=2.4188584057763718  RotationArbitraryAxis=[-0.6546536707079762 -0.37796447300923069 -0.65465367070797598]  FollAlignAxisA=+X  BaseAlignAxisA=+Y  FollAlignAxisB=+Y  BaseAlignAxisB=+Z  RotationSequenceAxes=FollowerAxes  RotationSequence=XYX  RotationSequenceAngles=[0 0 0]  RotationSequenceAnglesUnits=deg  RotationMatrix=[1 0 0; 0 1 0; 0 0 1]
  Transform53 : sm_lib/Frames and Transforms/Rigid Transform  TranslationMethod=None  TranslationStandardOffset=0  TranslationLengthUnit=m  TranslationStandardAxis=+Z  TranslationCartesianOffset=[0 0 0]  TranslationROffset=0  TranslationROffsetUnits=m  TranslationZOffset=0  TranslationZOffsetUnits=m  TranslationThetaOffset=0  TranslationThetaOffsetUnits=deg  RotationMethod=None  RotationAngleUnits=deg  RotationStandardAxis=+Z  RotationAngle=0  RotationArbitraryAxis=[0 0 1]  FollAlignAxisA=+X  BaseAlignAxisA=+Y  FollAlignAxisB=+Y  BaseAlignAxisB=+Z  RotationSequenceAxes=FollowerAxes  RotationSequence=XYX  RotationSequenceAngles=[0 0 0]  RotationSequenceAnglesUnits=deg  RotationMatrix=[1 0 0; 0 1 0; 0 0 1]
  Transform54 : sm_lib/Frames and Transforms/Rigid Transform  TranslationMethod=Cartesian  TranslationStandardOffset=200  TranslationLengthUnit=mm  TranslationStandardAxis=+Z  TranslationCartesianOffset=[-30 40 75]  TranslationROffset=0  TranslationROffsetUnits=m  TranslationZOffset=0  TranslationZOffsetUnits=m  TranslationThetaOffset=0  TranslationThetaOffsetUnits=deg  RotationMethod=None  RotationAngleUnits=rad  RotationStandardAxis=+Z  RotationAngle=0  RotationArbitraryAxis=[1 0 0]  FollAlignAxisA=+X  BaseAlignAxisA=+Y  FollAlignAxisB=+Y  BaseAlignAxisB=+Z  RotationSequenceAxes=FollowerAxes  RotationSequence=XYX  RotationSequenceAngles=[0 0 0]  RotationSequenceAnglesUnits=deg  RotationMatrix=[1 0 0; 0 1 0; 0 0 1]
  Transform6 : sm_lib/Frames and Transforms/Rigid Transform  TranslationMethod=Cartesian  TranslationStandardOffset=0  TranslationLengthUnit=mm  TranslationStandardAxis=+Z  TranslationCartesianOffset=[10.619396930206873 115.03911940923673 52.900000000000013]  TranslationROffset=0  TranslationROffsetUnits=m  TranslationZOffset=0  TranslationZOffsetUnits=m  TranslationThetaOffset=0  TranslationThetaOffsetUnits=deg  RotationMethod=ArbitraryAxis  RotationAngleUnits=rad  RotationStandardAxis=+Z  RotationAngle=3.1415926535897931  RotationArbitraryAxis=[0.98901586336191671 0.14780941112961193 -7.4147043167175484e-17]  FollAlignAxisA=+X  BaseAlignAxisA=+Y  FollAlignAxisB=+Y  BaseAlignAxisB=+Z  RotationSequenceAxes=FollowerAxes  RotationSequence=XYX  RotationSequenceAngles=[0 0 0]  RotationSequenceAnglesUnits=deg  RotationMatrix=[1 0 0; 0 1 0; 0 0 1]
  Transform7 : sm_lib/Frames and Transforms/Rigid Transform  TranslationMethod=Cartesian  TranslationStandardOffset=0  TranslationLengthUnit=mm  TranslationStandardAxis=+Z  TranslationCartesianOffset=[0.3122146831511497 36.930882126810701 38.499999999999979]  TranslationROffset=0  TranslationROffsetUnits=m  TranslationZOffset=0  TranslationZOffsetUnits=m  TranslationThetaOffset=0  TranslationThetaOffsetUnits=deg  RotationMethod=ArbitraryAxis  RotationAngleUnits=rad  RotationStandardAxis=+Z  RotationAngle=3.1415926535897927  RotationArbitraryAxis=[0.38719377190488019 -0.92199836388036582 -3.5277797665665267e-16]  FollAlignAxisA=+X  BaseAlignAxisA=+Y  FollAlignAxisB=+Y  BaseAlignAxisB=+Z  RotationSequenceAxes=FollowerAxes  RotationSequence=XYX  RotationSequenceAngles=[0 0 0]  RotationSequenceAnglesUnits=deg  RotationMatrix=[1 0 0; 0 1 0; 0 0 1]
  Transform8 : sm_lib/Frames and Transforms/Rigid Transform  TranslationMethod=Cartesian  TranslationStandardOffset=0  TranslationLengthUnit=mm  TranslationStandardAxis=+Z  TranslationCartesianOffset=[-5.1270705163374286 124.55210780981125 52.900000000000013]  TranslationROffset=0  TranslationROffsetUnits=m  TranslationZOffset=0  TranslationZOffsetUnits=m  TranslationThetaOffset=0  TranslationThetaOffsetUnits=deg  RotationMethod=ArbitraryAxis  RotationAngleUnits=rad  RotationStandardAxis=+Z  RotationAngle=3.1415926535897931  RotationArbitraryAxis=[0.36650122672429392 0.93041756798202591 2.9831310769236364e-17]  FollAlignAxisA=+X  BaseAlignAxisA=+Y  FollAlignAxisB=+Y  BaseAlignAxisB=+Z  RotationSequenceAxes=FollowerAxes  RotationSequence=XYX  RotationSequenceAngles=[0 0 0]  RotationSequenceAnglesUnits=deg  RotationMatrix=[1 0 0; 0 1 0; 0 0 1]
  Transform9 : sm_lib/Frames and Transforms/Rigid Transform  TranslationMethod=Cartesian  TranslationStandardOffset=0  TranslationLengthUnit=mm  TranslationStandardAxis=+Z  TranslationCartesianOffset=[-39.03991378494019 137.80425887104397 36.099999999999966]  TranslationROffset=0  TranslationROffsetUnits=m  TranslationZOffset=0  TranslationZOffsetUnits=m  TranslationThetaOffset=0  TranslationThetaOffsetUnits=deg  RotationMethod=ArbitraryAxis  RotationAngleUnits=rad  RotationStandardAxis=+Z  RotationAngle=1.6198107529808947  RotationArbitraryAxis=[0.21611670615757558 -0.95214869565588378 0.21611670615757447]  FollAlignAxisA=+X  BaseAlignAxisA=+Y  FollAlignAxisB=+Y  BaseAlignAxisB=+Z  RotationSequenceAxes=FollowerAxes  RotationSequence=XYX  RotationSequenceAngles=[0 0 0]  RotationSequenceAnglesUnits=deg  RotationMatrix=[1 0 0; 0 1 0; 0 0 1]
  Vis_tle_tte_cylindrique_cruciforme_H_29x13_C_10_RIGID : Subsystem
  Vis_tle_tte_cylindrique_cruciforme_H_29x13_C_11_RIGID : Subsystem
  Vis_tle_tte_cylindrique_cruciforme_H_29x13_C_12_RIGID : Subsystem
  Vis_tle_tte_cylindrique_cruciforme_H_29x13_C_13_RIGID : Subsystem
  Vis_tle_tte_cylindrique_cruciforme_H_29x13_C_14_RIGID : Subsystem
  Vis_tle_tte_cylindrique_cruciforme_H_29x13_C_15_RIGID : Subsystem
  Vis_tle_tte_cylindrique_cruciforme_H_29x13_C_16_RIGID : Subsystem
  Vis_tle_tte_cylindrique_cruciforme_H_29x13_C_17_RIGID : Subsystem
  Vis_tle_tte_cylindrique_cruciforme_H_29x13_C_18_RIGID : Subsystem
  Vis_tle_tte_cylindrique_cruciforme_H_29x13_C_19_RIGID : Subsystem
  Vis_tle_tte_cylindrique_cruciforme_H_29x13_C_1_RIGID : Subsystem
  Vis_tle_tte_cylindrique_cruciforme_H_29x13_C_20_RIGID : Subsystem
  Vis_tle_tte_cylindrique_cruciforme_H_29x13_C_21_RIGID : Subsystem
  Vis_tle_tte_cylindrique_cruciforme_H_29x13_C_22_RIGID : Subsystem
  Vis_tle_tte_cylindrique_cruciforme_H_29x13_C_23_RIGID : Subsystem
  Vis_tle_tte_cylindrique_cruciforme_H_29x13_C_2_RIGID : Subsystem
  Vis_tle_tte_cylindrique_cruciforme_H_29x13_C_3_RIGID : Subsystem
  Vis_tle_tte_cylindrique_cruciforme_H_29x13_C_4_RIGID : Subsystem
  Vis_tle_tte_cylindrique_cruciforme_H_29x13_C_5_RIGID : Subsystem
  Vis_tle_tte_cylindrique_cruciforme_H_29x13_C_7_RIGID : Subsystem
  Vis_tle_tte_cylindrique_cruciforme_H_29x13_C_8_RIGID : Subsystem
  Vis_tle_tte_cylindrique_cruciforme_H_29x13_C_9_RIGID : Subsystem
  Vis_tle_tte_cylindrique_cruciforme_H_29x8_C_1_RIGID : Subsystem
  Vis_tle_tte_cylindrique_cruciforme_H_29x8_C_2_RIGID : Subsystem
  Vis_tle_tte_cylindrique_cruciforme_H_29x8_C_3_RIGID : Subsystem
  carter_avant_1_RIGID : Subsystem
  carter_transparant_5_RIGID : Subsystem
  petite_carte_1_RIGID : Subsystem
  petite_carte_2_RIGID : Subsystem
  petite_carte_3_RIGID : Subsystem
  plaque_fixation_1_RIGID : Subsystem
  socle_1_RIGID : Subsystem
  vis_CHC_M4_30_1_RIGID : Subsystem
  vis_CHC_M4_30_2_RIGID : Subsystem
  F5 : PMIOPort  Side=Left
  F4 : PMIOPort  Port=2  Side=Right
  F3 : PMIOPort  Port=3  Side=Right
  F2 : PMIOPort  Port=4  Side=Right
  F1 : PMIOPort  Port=5  Side=Right
  F : PMIOPort  Port=6  Side=Right
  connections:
  Transform/LConn1 -- Transform54/LConn1 -- Transform8/LConn1 -- Transform9/LConn1 -- Transform7/LConn1 -- Transform6/LConn1 -- Transform53/LConn1 -- Transform52/LConn1 -- Transform51/LConn1 -- Transform50/LConn1 -- Transform5/LConn1 -- Transform49/LConn1 -- Transform48/LConn1 -- Transform47/LConn1 -- Transform46/LConn1 -- Transform45/LConn1 -- Transform44/LConn1 -- Transform43/LConn1 -- Transform42/LConn1 -- Transform41/LConn1 -- Transform40/LConn1 -- Transform4/LConn1 -- Transform39/LConn1 -- Transform38/LConn1 -- Transform37/LConn1 -- Transform36/LConn1 -- Transform35/LConn1 -- Transform34/LConn1 -- ReferenceFrame/RConn1 -- carter_avant_1_RIGID/RConn1 -- carter_transparant_5_RIGID/RConn1 -- F5/RConn1 -- Transform33/LConn1 -- Transform32/LConn1 -- Transform31/LConn1 -- Transform30/LConn1 -- Transform3/LConn1 -- Transform29/LConn1 -- Transform28/LConn1 -- Transform27/LConn1 -- Transform26/LConn1 -- Transform25/LConn1 -- Transform24/LConn1 -- Transform23/LConn1 -- Transform22/LConn1 -- Transform21/LConn1 -- Transform20/LConn1 -- Transform2/LConn1 -- Transform19/LConn1 -- Transform18/LConn1 -- Transform17/LConn1 -- Transform16/LConn1 -- Transform15/LConn1 -- Transform14/LConn1 -- Transform13/LConn1 -- Transform12/LConn1 -- Transform11/LConn1 -- Transform10/LConn1 -- Transform1/LConn1
  Transform/RConn1 -- F/RConn1
  Transform9/RConn1 -- Vis_tle_tte_cylindrique_cruciforme_H_29x13_C_11_RIGID/LConn1
  Transform10/RConn1 -- Vis_tle_tte_cylindrique_cruciforme_H_29x13_C_13_RIGID/LConn1
  Transform11/RConn1 -- Vis_tle_tte_cylindrique_cruciforme_H_29x13_C_9_RIGID/LConn1
  Transform12/RConn1 -- Vis_tle_tte_cylindrique_cruciforme_H_29x13_C_8_RIGID/LConn1
  Transform13/RConn1 -- Vis_tle_tte_cylindrique_cruciforme_H_29x8_C_3_RIGID/LConn1
  Transform14/RConn1 -- Vis_tle_tte_cylindrique_cruciforme_H_29x13_C_12_RIGID/LConn1
  Transform15/RConn1 -- Vis_tle_tte_cylindrique_cruciforme_H_29x13_C_10_RIGID/LConn1
  Rondelle_M4_2_RIGID/LConn1 -- Transform16/RConn1
  CARTE_HEXAGONALE_1_RIGID/LConn1 -- Transform17/RConn1
  Transform18/RConn1 -- Vis_tle_tte_cylindrique_cruciforme_H_29x13_C_5_RIGID/LConn1
  Transform1/RConn1 -- F1/RConn1
  Transform19/RConn1 -- petite_carte_1_RIGID/LConn1
  Transform20/RConn1 -- Vis_tle_tte_cylindrique_cruciforme_H_29x8_C_1_RIGID/LConn1
  FIXATION_MOTEUR_1_RIGID/LConn1 -- Transform21/RConn1
  FIXATION_MOTEUR_2_RIGID/LConn1 -- Transform22/RConn1
  Transform23/RConn1 -- Vis_tle_tte_cylindrique_cruciforme_H_29x13_C_1_RIGID/LConn1
  Transform24/RConn1 -- Vis_tle_tte_cylindrique_cruciforme_H_29x13_C_2_RIGID/LConn1
  Transform25/RConn1 -- Vis_tle_tte_cylindrique_cruciforme_H_29x13_C_3_RIGID/LConn1
  Transform26/RConn1 -- Vis_tle_tte_cylindrique_cruciforme_H_29x13_C_4_RIGID/LConn1
  Transform27/RConn1 -- socle_1_RIGID/LConn1
  Transform28/RConn1 -- vis_CHC_M4_30_1_RIGID/LConn1
  Transform2/RConn1 -- F2/RConn1
  Transform29/RConn1 -- vis_CHC_M4_30_2_RIGID/LConn1
  Rondelle_M4_1_RIGID/LConn1 -- Transform30/RConn1
  CARTER_ARRIERE_1_RIGID/LConn1 -- Transform31/RConn1
  Transform32/RConn1 -- Vis_tle_tte_cylindrique_cruciforme_H_29x13_C_18_RIGID/LConn1
  Transform33/RConn1 -- Vis_tle_tte_cylindrique_cruciforme_H_29x13_C_19_RIGID/LConn1
  Transform34/RConn1 -- Vis_tle_tte_cylindrique_cruciforme_H_29x13_C_20_RIGID/LConn1
  Transform35/RConn1 -- Vis_tle_tte_cylindrique_cruciforme_H_29x13_C_21_RIGID/LConn1
  Transform36/RConn1 -- Vis_tle_tte_cylindrique_cruciforme_H_29x13_C_22_RIGID/LConn1
  Transform37/RConn1 -- Vis_tle_tte_cylindrique_cruciforme_H_29x13_C_23_RIGID/LConn1
  FIXATION_MOTEUR_5_RIGID/LConn1 -- Transform38/RConn1
  Transform3/RConn1 -- F3/RConn1
  FIXATION_MOTEUR_6_RIGID/LConn1 -- Transform39/RConn1
  PLAQUE_NOM_1_RIGID/LConn1 -- Transform40/RConn1
  CACHE_1_RIGID/LConn1 -- Transform41/RConn1
  CACHE_2_RIGID/LConn1 -- Transform42/RConn1
  CACHE_3_RIGID/LConn1 -- Transform43/RConn1
  Transform44/RConn1 -- Vis_tle_tte_cylindrique_cruciforme_H_29x13_C_7_RIGID/LConn1
  Transform45/RConn1 -- Vis_tle_tte_cylindrique_cruciforme_H_29x13_C_14_RIGID/LConn1
  Transform46/RConn1 -- Vis_tle_tte_cylindrique_cruciforme_H_29x13_C_15_RIGID/LConn1
  MOTEUR_2_RIGID/LConn1 -- Transform47/RConn1
  MOTEUR_3_RIGID/LConn1 -- Transform48/RConn1
  Transform4/RConn1 -- F4/RConn1
  FIXATION_MOTEUR_3_RIGID/LConn1 -- Transform49/RConn1
  FIXATION_MOTEUR_4_RIGID/LConn1 -- Transform50/RConn1
  Transform51/RConn1 -- Vis_tle_tte_cylindrique_cruciforme_H_29x13_C_16_RIGID/LConn1
  Transform52/RConn1 -- Vis_tle_tte_cylindrique_cruciforme_H_29x13_C_17_RIGID/LConn1
  Transform53/RConn1 -- plaque_fixation_1_RIGID/LConn1
  Transform5/RConn1 -- Vis_tle_tte_cylindrique_cruciforme_H_29x8_C_2_RIGID/LConn1
  Transform6/RConn1 -- petite_carte_2_RIGID/LConn1
  MOTEUR_1_RIGID/LConn1 -- Transform7/RConn1
  Transform8/RConn1 -- petite_carte_3_RIGID/LConn1
  PLAQUE_NOM_SET/LConn1 -- Transform54/RConn1
